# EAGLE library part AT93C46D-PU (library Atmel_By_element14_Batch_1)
Three-wire Serial EEPROM
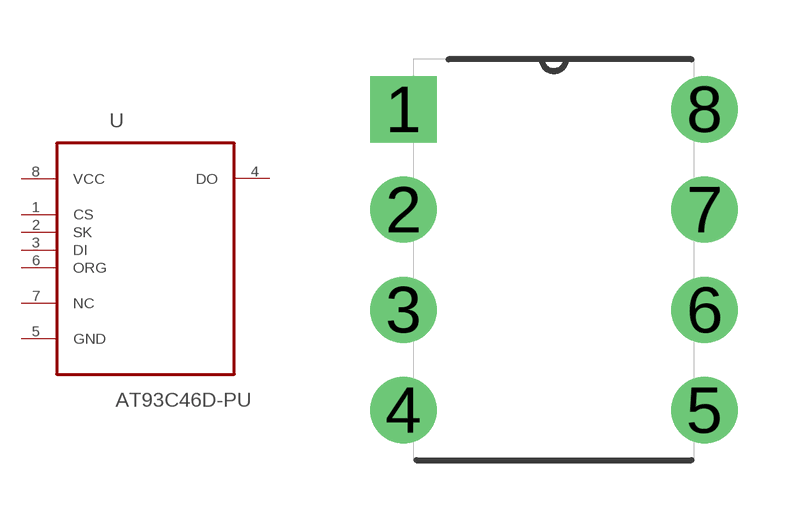
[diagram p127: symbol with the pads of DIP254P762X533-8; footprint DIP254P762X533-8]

Designator prefix U

## AT93C46D-PU (MPN: AT93C46D-PU; OC_FARNELL: 1362666; OC_NEWARK: 50M3339; PACKAGE: PDIP-8; SUPPLIER: Atmel)  [DIP254P762X533-8]
1  CS  in
2  SK  in
3  DI  in
4  DO  out
5  GND  pas
6  ORG  pas
7  NC  nc
8  VCC  pwr

## Footprint DIP254P762X533-8 (pad centres in mm)
drill 1.118 square: 1 -7.62,7.62
drill 1.118: 2 -7.62,5.08; 3 -7.62,2.54; 4 -7.62,0; 5 0,0; 6 0,2.54; 7 0,5.08; 8 0,7.62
